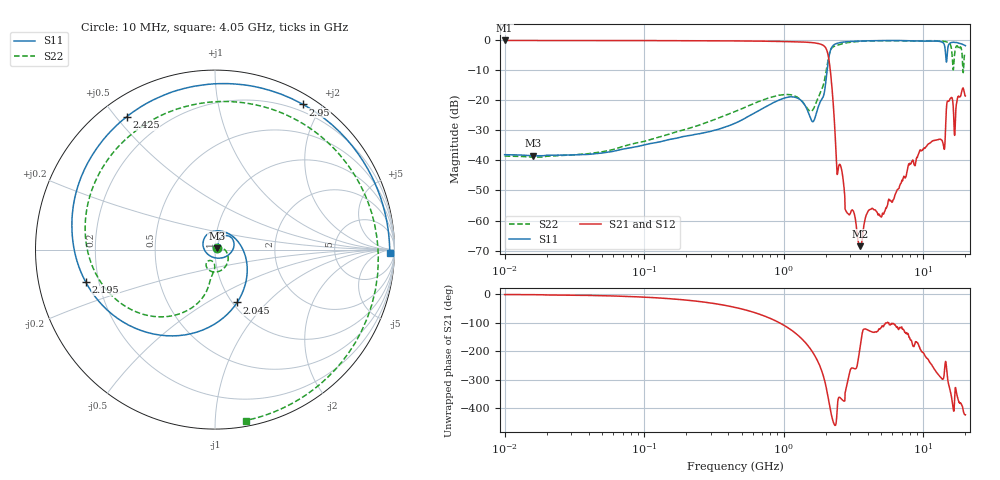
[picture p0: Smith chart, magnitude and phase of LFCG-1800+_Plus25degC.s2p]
! Mini-Circuits
! S2P DATA File Format
! Type: LOW PASS FILTER
! Model: LFCG-1800+
! All S Parameters are in dB deg format
! TEST CONDITIONS: INPUT POWER = 0 dBm @ Temperature = +25deg C
!S2P File: Measurements: S11, S21, S12, S22:
# Hz S  dB  R 50
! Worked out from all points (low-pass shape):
!   718 points, 10 MHz to 20 GHz, reference 50 ohm
!   highest |S21| = -0.12 dB at 10 MHz (marker M1); lowest = -68.5 dB at 3.5 GHz (marker M2)
!   |S21| within 3 dB of the highest: start of sweep to 2.023 GHz
!   lowest |S11| = -38.5 dB at 16 MHz (marker M3), VSWR 1.02, Z = 51 + j0.64 ohm
!   |S11| at or under -10 dB: start of sweep to 2.044 GHz
!   |S22| runs from -38.9 to -0.1 dB; largest |S21 - S12| = 0.00068
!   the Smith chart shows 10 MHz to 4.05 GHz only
!   S11 on the Smith chart (normalised r, x): 10 MHz: 1.02, +0.02; 2.045 GHz: 1.05, -0.69; 2.195 GHz: 0.15, -0.12; 2.425 GHz: 0.08, +0.53; 2.95 GHz: 0.11, +1.77; 4.05 GHz: 48, -36
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1e7  -38.10 42.7  -0.12 -1.5  -0.11 -1.5  -38.56 41.0
1.6e7  -38.47 31.7  -0.12 -1.9  -0.12 -1.9  -38.93 34.2
4e7  -37.99 31.1  -0.13 -4.5  -0.13 -4.5  -37.75 30.6
1.3e8  -33.81 43.5  -0.17 -13.7  -0.17 -13.7  -32.13 29.2
4.5e8  -27.59 63.6  -0.27 -46.8  -0.26 -46.8  -23.70 -11.4
1.02e9  -19.22 42.1  -0.48 -111.3  -0.48 -111.3  -18.06 -87.0
1.59e9  -26.94 -96.2  -0.82 160.6  -0.82 160.6  -23.55 -103.1
1.865e9  -19.81 94.6  -1.47 92.5  -1.47 92.5  -16.55 -97.0
2.045e9  -9.92 -67.2  -3.74 16.4  -3.74 16.4  -8.13 -116.8
2.195e9  -2.58 -165.9  -13.84 -63.6  -13.85 -63.6  -2.79 174.3
2.425e9  -1.02 123.6  -44.53 -27.2  -44.54 -27.2  -1.69 90.4
2.95e9  -0.48 58.7  -58.13 81.4  -58.10 81.3  -0.76 -8.1
3.5e9  -0.31 22.6  -68.52 165.0  -68.52 164.6  -0.42 -54.7
4.05e9  -0.23 -1.2  -56.65 -127.0  -56.65 -127.2  -0.29 -79.8
5.65e9  -0.13 -38.1  -52.88 -100.3  -52.88 -100.4  -0.19 -117.3
9.15e9  -0.32 -76.8  -38.32 -172.9  -38.32 -172.9  -0.24 180.0
1.215e10  -0.29 -108.9  -33.31 92.9  -33.31 92.8  -0.21 121.0
1.41e10  -1.43 -167.2  -36.33 80.9  -36.33 80.9  -0.42 89.3
1.59e10  -0.80 159.5  -19.06 0.1  -19.06 0.1  -2.97 31.9
1.635e10  -0.71 148.6  -21.91 -41.4  -21.91 -41.5  -9.89 -86.6
1.675e10  -0.76 141.5  -31.67 -6.8  -31.68 -6.9  -4.47 156.3
2e10  -1.86 121.1  -18.58 -62.7  -18.58 -62.8  -4.35 113.4
